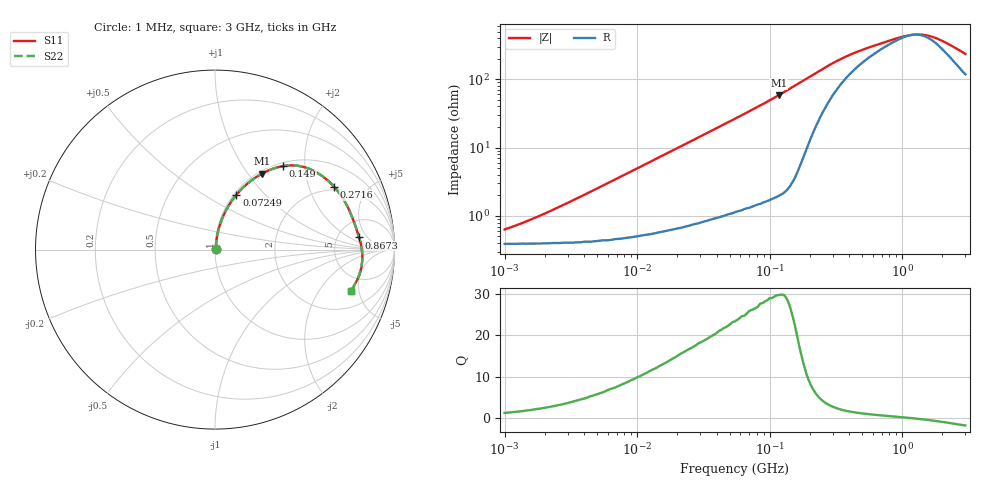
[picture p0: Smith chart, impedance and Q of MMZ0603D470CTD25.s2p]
! S-Parameter Data Generated by TDK Corporation
! Copyright(C) 2025 TDK Corporation.
! All Rights Reserved.
! TDK P/N: MMZ0603D470CTD25 (Chip Bead)
! Property: |Z|=47ohm at 100MHz
! Size(LxWxT): 0.6x0.3x0.3mm
! Model Type: s2p (Touchstone File Format Version 1.0)
! Frequency: DC=Yes Start=1MHz Stop=3000MHz 202points Log-sweep
! Model Generated on Feb. 6, 2025
! Terms and conditions regarding TDK Simulation Models:
! 1)This simulation model is being provided solely for informational
!  purposes. Please refer to the specifications of the products in
!  terms of detailed characteristics of such products.
! 2)In no event shall TDK Corporation of any of its subsidiaries be
!  liable for any loss or damage arising, directly or indirectly,
!  from any information contained in this simulation model, including,
!  but not limited to loss or damages arising from any inaccuracies,
!  omissions or errors in connection with such information.
! 3)Any and all copyrights on this simulation model are owned by
!  TDK Corporation.  Duplication or redistribution of this simulation
!  model without prior written permission from TDK Corporation
!  is prohibited.
! 4)This simulation model is subject to any modification or change
!  without any prior notice.
! 5)Neither TDK Corporation nor any of its subsidiaries shall make any
!  warranty, express or implied, including but not limited to the
!  correctness, implied warranties of merchantability and fitness for
!  a particular purpose with respect to this simulation models.
! 6)The use of this simulation model shall be deemed to have consented
!  to the terms and conditions hereof.
! Port Assignments:
!  1 ---@@@--- 2
! Applicable Conditions:
!  Temperature = 25 degC
!  DC Bias Current = 0 A
!  Small Signal Operation
# Hz S MA R 50
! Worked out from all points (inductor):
!   201 points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, 1 MHz to 3 GHz, reference 50 ohm
!   read as one part in series: L = 79.8 nH near 2.413 MHz
!   highest Q = 29.7 at 117.2 MHz (marker M1), where L = 79.5 nH
!   self-resonance near 1.219 GHz
!   S11 on the Smith chart (normalised r, x): 1 MHz: 1.01, +0.01; 72.49 MHz: 1.03, +0.70; 149 MHz: 1.06, +1.54; 271.6 MHz: 1.86, +2.98; 867.3 MHz: 8.09, +3.12; 3 GHz: 3.37, -4.07
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1000000  0.006311 51.8  0.9961 -0.3  0.9961 -0.3  0.006311 51.8
1751453  0.009589 65.3  0.996 -0.5  0.996 -0.5  0.009589 65.3
3900413  0.01984 76.8  0.9957 -1.1  0.9957 -1.1  0.01984 76.8
1.461624e7  0.07139 81.4  0.9918 -4.1  0.9918 -4.1  0.07139 81.4
3.00453e7  0.1433 78.6  0.9819 -8.2  0.9819 -8.2  0.1433 78.6
5.477226e7  0.2534 72.9  0.9566 -14.7  0.9566 -14.7  0.2534 72.9
7.248696e7  0.3278 68.7  0.9322 -19.1  0.9322 -19.1  0.3278 68.7
9.216659e7  0.4058 64.0  0.8996 -23.9  0.8996 -23.9  0.4058 64.0
1.171891e8  0.498 58.2  0.8506 -29.8  0.8506 -29.8  0.498 58.2
1.49005e8  0.5998 50.9  0.7762 -36.8  0.7762 -36.8  0.5998 50.9
1.748812e8  0.66 44.9  0.7079 -41.2  0.7079 -41.2  0.66 44.9
2.136344e8  0.7126 36.9  0.6065 -44.8  0.6065 -44.8  0.7126 36.9
2.716345e8  0.7507 27.7  0.4844 -46.2  0.4844 -46.2  0.7507 27.7
3.318279e8  0.7681 21.6  0.4018 -44.7  0.4018 -44.7  0.7681 21.6
4.0536e8  0.7787 16.8  0.3393 -41.4  0.3393 -41.4  0.7787 16.8
8.005644e8  0.8027 5.9  0.2176 -22.2  0.2176 -22.2  0.8027 5.9
8.672962e8  0.806 4.8  0.208 -18.9  0.208 -18.9  0.806 4.8
1.194682e9  0.8175 0.3  0.1826 -1.4  0.1826 -1.4  0.8175 0.3
1.519029e9  0.8224 -3.5  0.186 15.6  0.186 15.6  0.8224 -3.5
1.931433e9  0.8203 -7.7  0.2171 30.5  0.2171 30.5  0.8203 -7.7
2.359433e9  0.8118 -11.6  0.2621 38.6  0.2621 38.6  0.8118 -11.6
3e9  0.7887 -16.8  0.3348 43.0  0.3348 43.0  0.7887 -16.8
